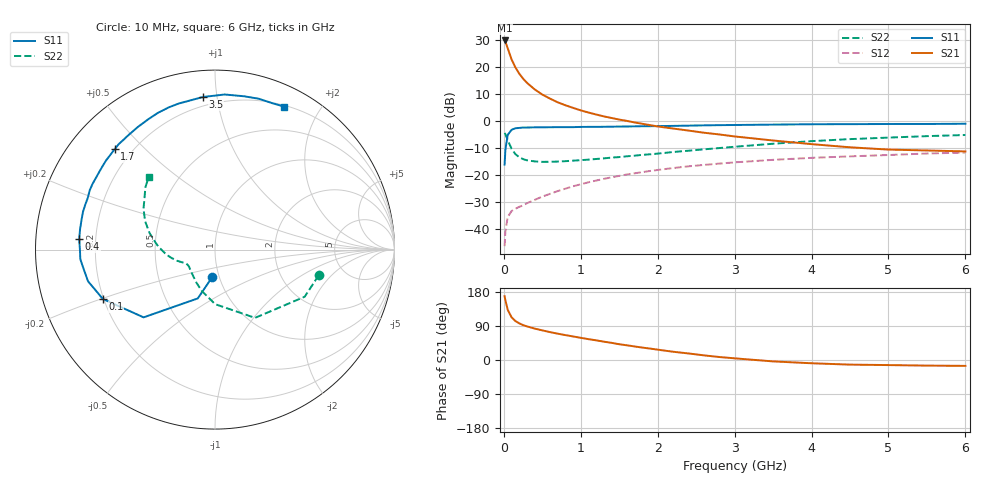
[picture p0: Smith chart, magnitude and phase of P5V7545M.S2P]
! SIEMENS Small Signal Semiconductors
! BFP183
! Si NPN RF Bipolar Junction Transistor in SOT143
! VCE = 0.75 V  IC = 45 mA
! Common Emitter S-Parameters:  March  1996
# GHz  S  MA  R  50
!  f  S11  S21  S12  S22
! GHz  MAG  ANG  MAG  ANG  MAG  ANG  MAG  ANG
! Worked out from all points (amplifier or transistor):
!   36 points, 10 MHz to 6 GHz, reference 50 ohm
!   highest |S21| = 29.9 dB at 10 MHz (marker M1)
!   |S21| within 3 dB of that: start of sweep to 51.57 MHz
!   unconditionally stable (mu >= 1): start of sweep to 27.91 MHz; 156.2 MHz to end of sweep
!   at 250 MHz: K = 1.32, MAG = 20.2 dB, |S12| = -31.4 dB
!   at 1.4 GHz: K = 1.98, MAG = 5.4 dB, |S12| = -21.0 dB
!   at 6 GHz: K = 1.55, MAG = -4.2 dB, |S12| = -11.8 dB
!   S11 on the Smith chart (normalised r, x): 10 MHz: 0.93, -0.29; 100 MHz: 0.20, -0.20; 400 MHz: 0.14, +0.04; 1.7 GHz: 0.14, +0.41; 3.5 GHz: 0.15, +0.91; 6 GHz: 0.21, +1.57
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0.01  0.154 -95.8  31.22 168.4  0.0047 64.2  0.5955 -13.9
0.02  0.2883 -109.4  29.62 157.5  0.0089 64.8  0.5645 -27.7
0.05  0.5484 -136.5  22.43 132.7  0.0163 50.0  0.441 -59.6
0.1  0.6824 -156.2  13.94 112.8  0.0211 38.9  0.3039 -89.9
0.15  0.7291 -166.0  9.86 102.9  0.0233 38.6  0.2412 -107.9
0.2  0.74 -171.7  7.549 96.8  0.0253 39.5  0.2111 -119.4
0.25  0.7524 -176.0  6.101 92.1  0.0269 41.7  0.1947 -127.3
0.3  0.7522 -179.4  5.106 88.7  0.0295 45.1  0.1851 -133.6
0.4  0.7588 175.6  3.852 82.9  0.034 49.0  0.1768 -141.7
0.5  0.7603 171.5  3.083 78.2  0.0392 51.8  0.1733 -146.3
0.6  0.7619 167.5  2.592 73.6  0.0441 53.9  0.1738 -149.6
0.7  0.765 164.0  2.215 69.5  0.0496 55.6  0.1755 -152.1
0.9  0.765 158.0  1.745 62.2  0.061 56.7  0.1825 -155.1
1.1  0.7742 151.8  1.43 55.0  0.0723 56.6  0.1906 -157.7
1.3  0.777 145.9  1.212 48.4  0.0838 55.9  0.2014 -159.9
1.7  0.7911 134.9  0.935 35.7  0.1062 52.4  0.2259 -164.9
2.2  0.8072 122.2  0.721 21.8  0.1329 46.9  0.264 -172.7
2.8  0.8332 108.0  0.56 7.9  0.1608 39.4  0.3128 177.6
3.5  0.8529 94.5  0.432 -3.7  0.1889 31.0  0.3761 165.8
4.5  0.8694 79.3  0.323 -12.2  0.219 19.6  0.4586 150.3
5.5  0.876 68.7  0.282 -14.8  0.2477 9.6  0.5208 138.1
6  0.8849 64.2  0.271 -15.5  0.2577 4.4  0.5468 132.6
